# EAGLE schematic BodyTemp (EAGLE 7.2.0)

## Sheet 1 of 4: nordic
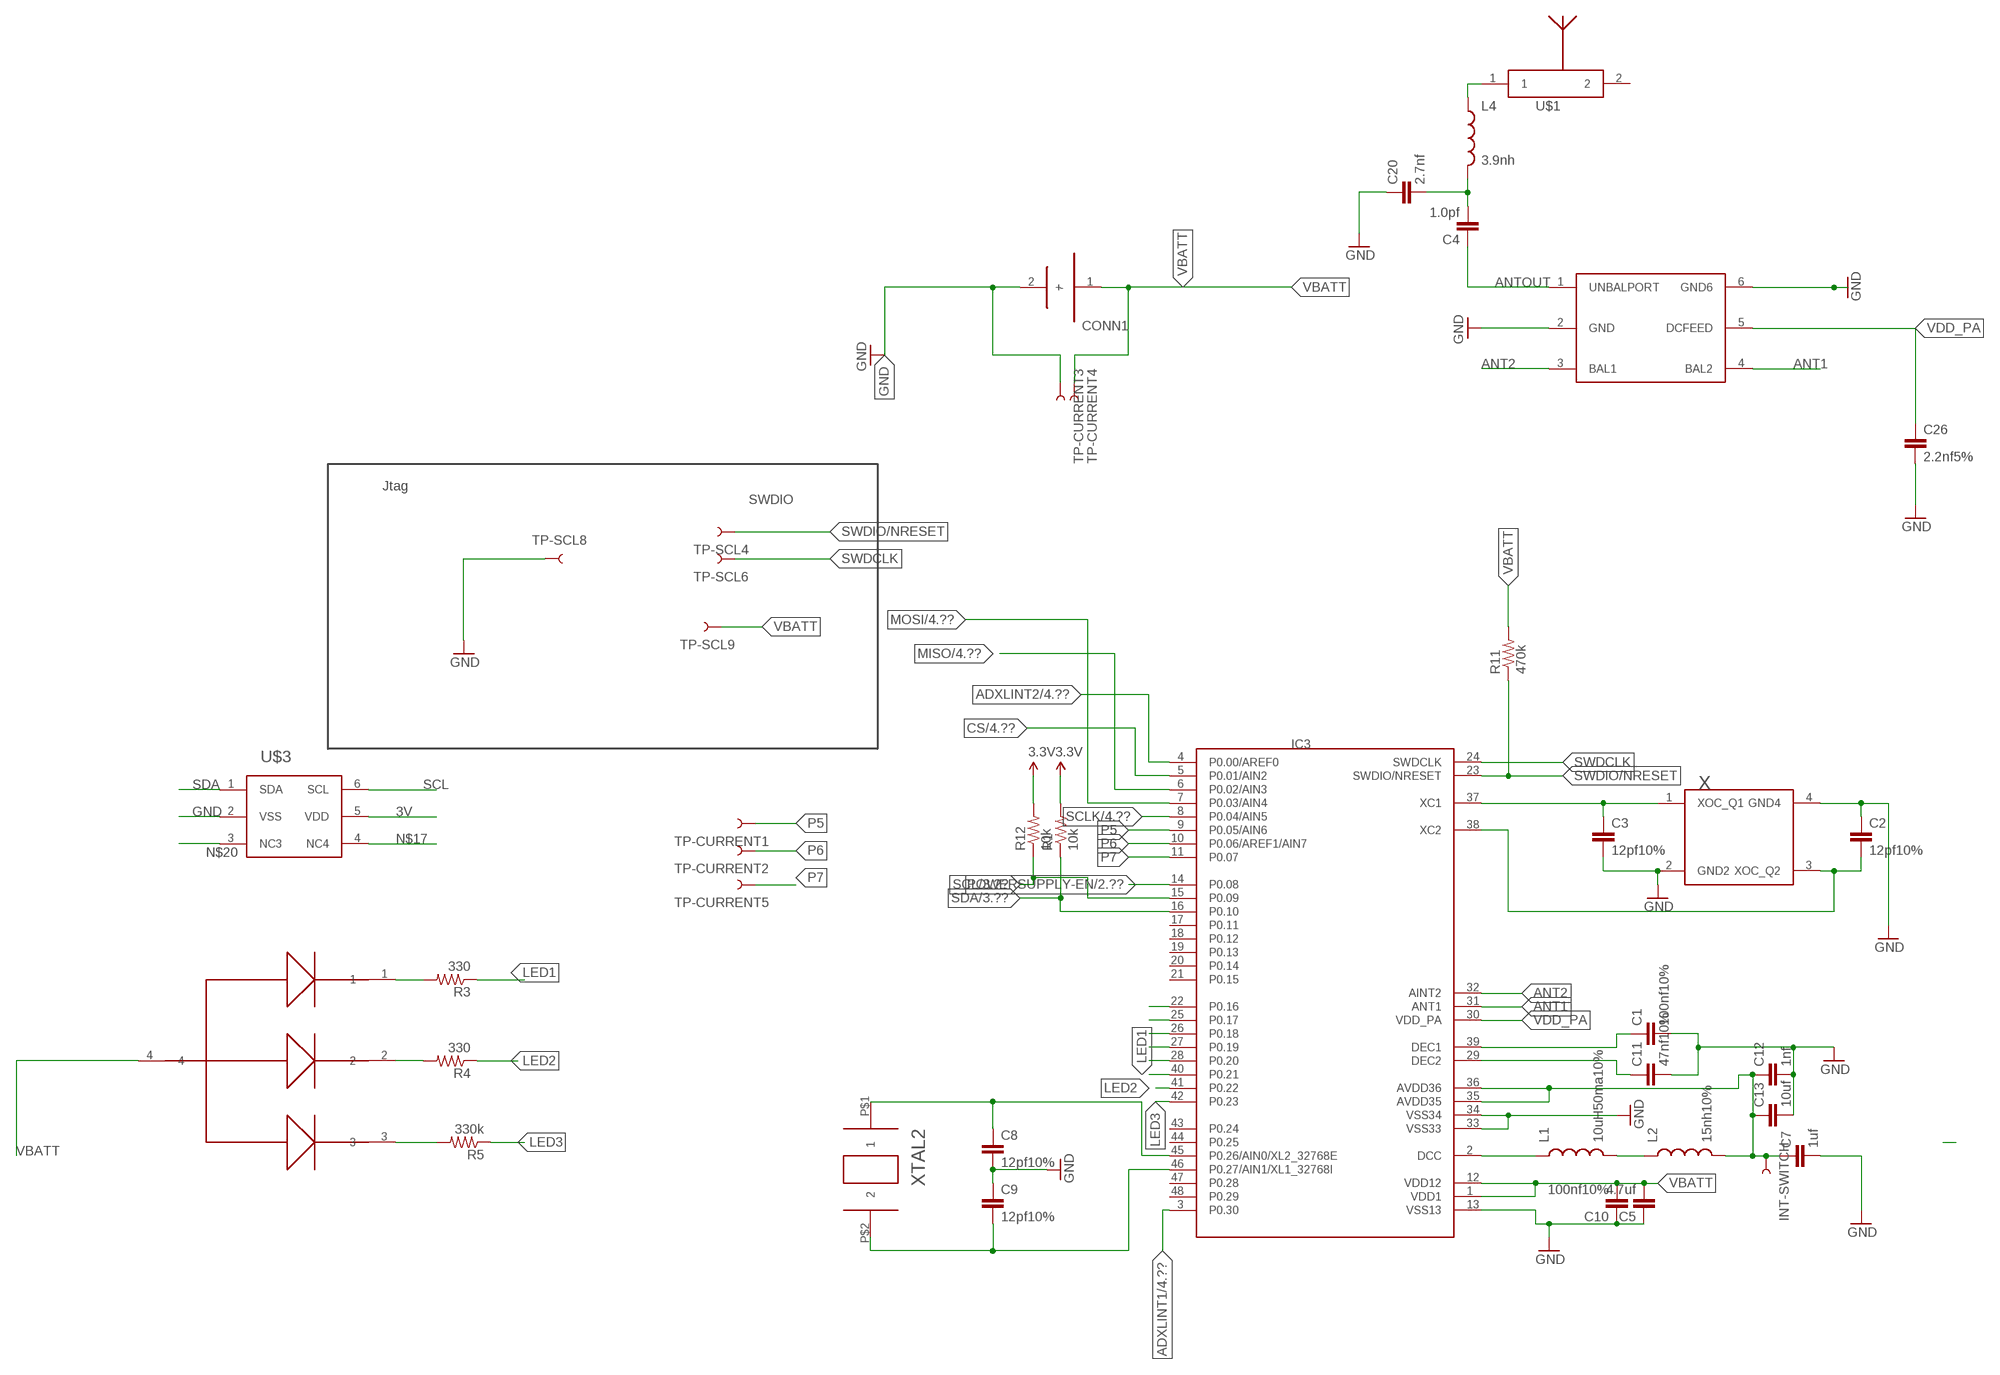
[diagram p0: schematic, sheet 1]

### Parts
C1  100nf10%  CAP0402-CAP  [0402-CAP]
C2  12pf10%  CAP0402-CAP  [0402-CAP]
C3  12pf10%  CAP0402-CAP  [0402-CAP]
C4  1.0pf  CAP0402-CAP  [0402-CAP]
C5  4.7uf  CAP0402-CAP  [0402-CAP]
C7  1uf  CAP0402-CAP  [0402-CAP]
C8  12pf10%  CAP0402-CAP  [0402-CAP]
C9  12pf10%  CAP0402-CAP  [0402-CAP]
C10  100nf10%  CAP0402-CAP  [0402-CAP]
C11  47nf10%  CAP0402-CAP  [0402-CAP]
C12  1nf  CAP0402-CAP  [0402-CAP]
C13  10uf  CAP0402-CAP  [0402-CAP]
C20  2.7nf  CAP0402-CAP  [0402-CAP]
C26  2.2nf5%  CAP0402-CAP  [0402-CAP]
CONN1  BATTHOLDER-ONBOARD  [BATTHOLDER-ONBOARD]
FILTER1  BAKUN-BPFILTER  [BALUN-PROTOTYPE]
IC3  NRF51  [QFN48(6MM-6MM)]
INT-SWITCH  TEST-POINT3  [PAD.03X.03]
L1  10uH50ma10%  INDUCTOR0603  [0603]
L2  15nh10%  INDUCTOR0402  [C0402]
L4  3.9nh  INDUCTOR0402  [C0402]
LED1  RGB-LED  [RGB-LTST-C19FD1WT]
R1  10k  RESISTOR0402-RES  [0402-RES]
R3  330  RESISTOR0402-RES  [0402-RES]
R4  330  RESISTOR0402-RES  [0402-RES]
R5  330k  RESISTOR0402-RES  [0402-RES]
R11  470k  RESISTOR0402-RES  [0402-RES]
R12  10k  RESISTOR0402-RES  [0402-RES]
TP-CURRENT1  TEST-POINT3  [PAD.03X.03]
TP-CURRENT2  TEST-POINT3  [PAD.03X.03]
TP-CURRENT3  TEST-POINT3  [PAD.03X.03]
TP-CURRENT4  TEST-POINT3  [PAD.03X.03]
TP-CURRENT5  TEST-POINT3  [PAD.03X.03]
TP-SCL4  TEST-POINT3  [PAD.03X.03]
TP-SCL6  TEST-POINT3  [PAD.03X.03]
TP-SCL8  TEST-POINT3  [PAD.03X.03]
TP-SCL9  TEST-POINT3  [PAD.03X.03]
U$1  2.4GHZ-CHIP-ANTENNA  [2.4GHZ-2450AT18A100]
U$3  STS21  [STS21]
X  XTAL16MHZ  [NX322DSA-16MHZ-T1]
XTAL2  XTAL32768KHZ  [TF20D]

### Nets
3V: R1.2 R12.2 U$3.5(VDD) ; supply symbol labelled 3.3V ; also sheet 2,3
32K_1: C8.1 IC3.45(P0.26/AIN0/XL2_32768E) XTAL2.P$1
32K_2: C9.2 IC3.46(P0.27/AIN1/XL1_32768I) XTAL2.P$2
ADXLINT1: IC3.3(P0.30) ; also sheet 4
ADXLINT2: IC3.4(P0.00/AREF0) ; also sheet 4
ANT1: FILTER1.4(BAL2) IC3.31(ANT1)
ANT2: FILTER1.3(BAL1) IC3.32(AINT2)
ANTOUT: C4.1 FILTER1.1(UNBALPORT)
AVDD: C7.1 C12.1 C13.1 IC3.35(AVDD35) IC3.36(AVDD36) INT-SWITCH.P$1 L2.2
CS: IC3.5(P0.01/AIN2) ; also sheet 4
GND: C1.2 C2.1 C3.2 C5.1 C7.2 C8.2 C9.1 C10.1 C11.2 C12.2 C13.2 C20.1 C26.2 CONN1.2(-) FILTER1.2(GND) FILTER1.6(GND6) IC3.13(VSS13) IC3.33(VSS33) IC3.34(VSS34) TP-CURRENT3.P$1 TP-SCL8.P$1 U$3.2(VSS) X.2(GND2) X.4(GND4) ; also sheet 2,3,4
LED1: IC3.40(P0.21) R3.1
LED2: IC3.41(P0.22) R4.1
LED3: IC3.42(P0.23) R5.1
MISO: IC3.6(P0.02/AIN3) ; also sheet 4
MOSI: IC3.7(P0.03/AIN4) ; also sheet 4
N$1: C3.1 IC3.37(XC1) X.1(XOC_Q1)
N$2: C2.2 IC3.38(XC2) X.3(XOC_Q2)
N$3: IC3.2(DCC) L1.1
N$4: L1.2 L2.1
N$6: C1.1 IC3.39(DEC1)
N$7: C11.1 IC3.29(DEC2)
N$11: LED1.1 R3.2
N$12: LED1.2 R4.2
N$13: L4.1 U$1.1
N$14: C4.2 C20.2 L4.2
N$15: LED1.3 R5.2
N$17: U$3.4(NC4)
N$19: IC3.22(P0.16)
N$20: U$3.3(NC3)
N$21: IC3.25(P0.17)
N$22: IC3.27(P0.19)
N$23: IC3.26(P0.18)
N$24: IC3.28(P0.20)
P5: IC3.9(P0.05/AIN6) TP-CURRENT1.P$1
P6: IC3.10(P0.06/AREF1/AIN7) TP-CURRENT2.P$1
P7: IC3.11(P0.07) TP-CURRENT5.P$1
POWERSUPPLY-EN: IC3.14(P0.08) ; also sheet 2
SCL: IC3.15(P0.09) R12.1 U$3.6(SCL) ; also sheet 3
SCLK: IC3.8(P0.04/AIN5) ; also sheet 4
SDA: IC3.16(P0.10) R1.1 U$3.1(SDA) ; also sheet 3
SWDCLK: IC3.24(SWDCLK) TP-SCL6.P$1
SWDIO/NRESET: IC3.23(SWDIO/NRESET) R11.1 TP-SCL4.P$1
VBATT: C5.2 C10.2 CONN1.1(+) IC3.1(VDD1) IC3.12(VDD12) LED1.4 R11.2 TP-CURRENT4.P$1 TP-SCL9.P$1 ; also sheet 4
VDD_PA: C26.1 FILTER1.5(DCFEED) IC3.30(VDD_PA)
Unconnected: IC3.17(P0.11) IC3.18(P0.12) IC3.19(P0.13) IC3.20(P0.14) IC3.21(P0.15) IC3.43(P0.24) IC3.44(P0.25) IC3.47(P0.28) IC3.48(P0.29) U$1.2

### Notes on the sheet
- Jtag
- SWDIO

## Sheet 2 of 4: 3.3volts
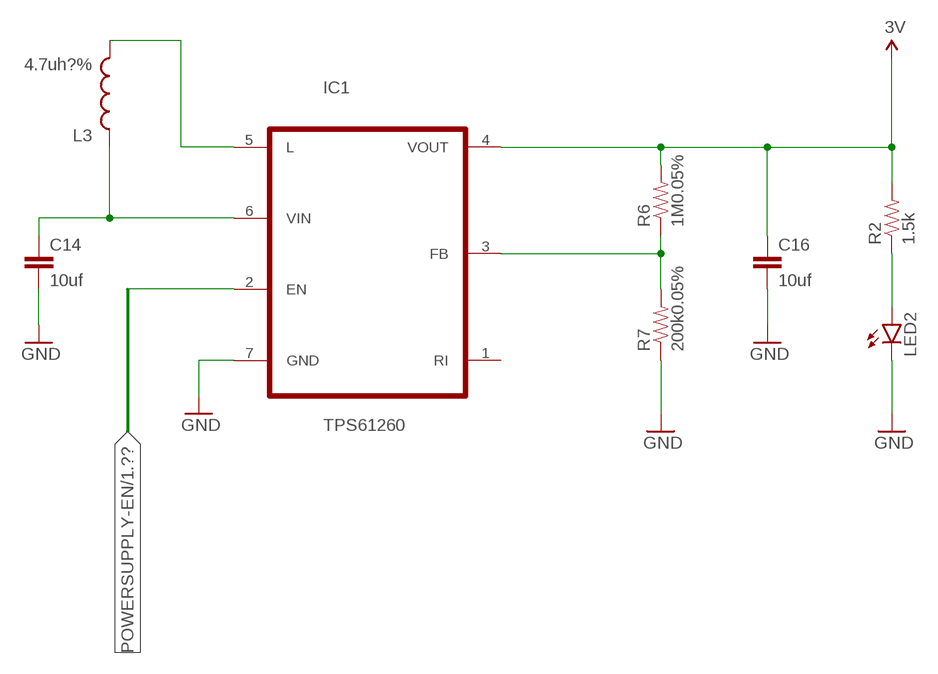
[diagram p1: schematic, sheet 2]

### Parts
C14  10uf  CAP0402-CAP  [0402-CAP]
C16  10uf  CAP0402-CAP  [0402-CAP]
IC1  TPS61260  [TP61260]
L3  4.7uh?%  INDUCTOR0805  [0805]
LED2  LED0603  [LED-0603]
R2  1.5k  RESISTOR0402-RES  [0402-RES]
R6  1M0.05%  RESISTOR0402-RES  [0402-RES]
R7  200k0.05%  RESISTOR0402-RES  [0402-RES]

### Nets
3V: C16.1 IC1.4(VOUT) R2.2 R6.2 ; also sheet 1,3
GND: C14.2 C16.2 IC1.7(GND) LED2.C R7.1 ; also sheet 1,3,4
N$5: IC1.5(L) L3.2
N$8: IC1.3(FB) R6.1 R7.2
N$9: C14.1 IC1.6(VIN) L3.1
N$10: LED2.A R2.1
POWERSUPPLY-EN: IC1.2(EN) ; also sheet 1
Unconnected: IC1.1(RI)

## Sheet 3 of 4: mlx
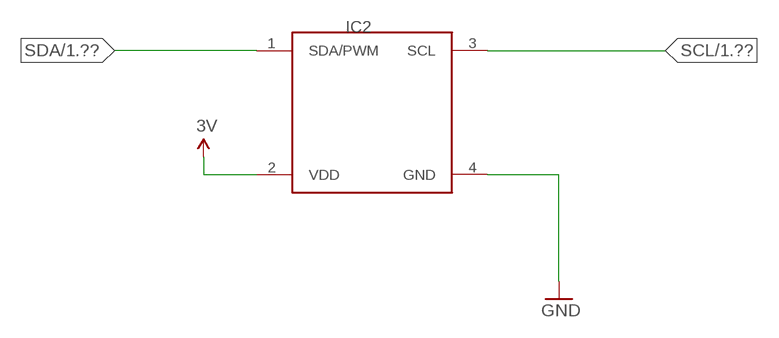
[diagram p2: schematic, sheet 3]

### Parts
IC2  MLX90615  [TO-46]

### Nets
3V: IC2.2(VDD) ; also sheet 1,2
GND: IC2.4(GND) ; also sheet 1,2,4
SCL: IC2.3(SCL) ; also sheet 1
SDA: IC2.1(SDA/PWM) ; also sheet 1

## Sheet 4 of 4: adxl362
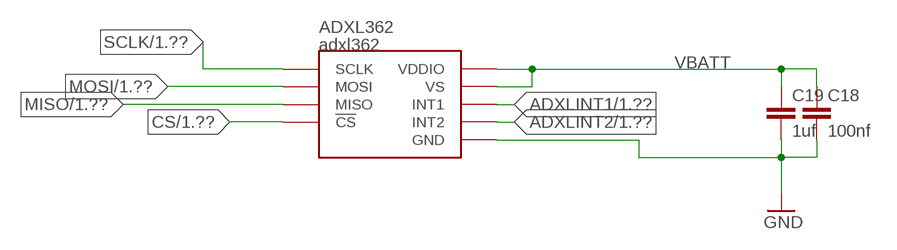
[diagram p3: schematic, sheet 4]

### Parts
ADXL362  adxl362  ADXL362ADXL362-1:1  [ADXL362-1:1]
C18  100nf  CAP0402-CAP  [0402-CAP]
C19  1uf  CAP0402-CAP  [0402-CAP]

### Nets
ADXLINT1: ADXL362.P$11(INT1) ; also sheet 1
ADXLINT2: ADXL362.P$9(INT2) ; also sheet 1
CS: ADXL362.P$8(!CS) ; also sheet 1
GND: ADXL362.P$12(GND) ADXL362.P$13(GND) ADXL362.P$16(GND) C18.2 C19.2 ; also sheet 1,2,3
MISO: ADXL362.P$7(MISO) ; also sheet 1
MOSI: ADXL362.P$6(MOSI) ; also sheet 1
SCLK: ADXL362.P$4(SCLK) ; also sheet 1
VBATT: ADXL362.P$1(VDDIO) ADXL362.P$14(VS) C18.1 C19.1 ; also sheet 1

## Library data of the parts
ADXL362 = SparkFun-Sensors:ADXL362: Micropower 3-axis accelerometer 2/4/8g digital output (SPI) IC-11297
C1-C5 C7-C14 C16 C18-C20 C26 = BodyTemp:CAP: Capacitor
CONN1 = BodyTemp:BATTHOLDER-ONBOARD
FILTER1 = BodyTemp:BAKUN-BPFILTER
IC1 = BodyTemp:TPS61260
IC2 = BodyTemp:MLX90615
IC3 = BodyTemp:NRF51
INT-SWITCH TP-CURRENT1-TP-CURRENT5 TP-SCL4 TP-SCL6 TP-SCL8 TP-SCL9 = SparkFun-Passives:TEST-POINT: Bare copper test points for troubleshooting or ICT
L1-L4 = BodyTemp:INDUCTOR: Inductors
LED1 = BodyTemp:RGB-LED
LED2 = BodyTemp:LED: LEDs
R1-R7 R11 R12 = BodyTemp:RESISTOR: Resistor
U$1 = BodyTemp:2.4GHZ-CHIP-ANTENNA
U$3 = BodyTemp:STS21
X = BodyTemp:XTAL16MHZ
XTAL2 = BodyTemp:XTAL32768KHZ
